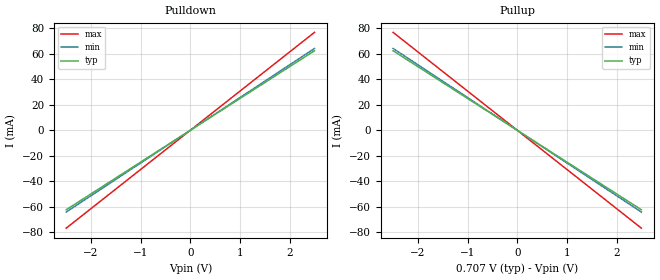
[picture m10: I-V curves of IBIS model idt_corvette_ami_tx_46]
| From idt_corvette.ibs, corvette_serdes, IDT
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|   model   idt_corvette_ami_tx_46
[Model] idt_corvette_ami_tx_46
Model_type Output
C_comp 400f 400f 400f
Cref = 0
[Model Spec]
Vmeas 0. 0. 0.
Vref 0. 0. 0.
[Temperature Range]  25 100 0
[Voltage Range] .707 .697 .631
[Algorithmic Model]
Executable Windows_VisualStudio5_32 idt_corvette_tx.dll   idt_corvette_tx.ami
Executable Windows_ver_64   idt_corvette_tx_64.dll   idt_corvette_tx.ami
Executable Linux_gcc4.1.2_32   idt_corvette_tx.linux.so   idt_corvette_tx.ami
Executable Linux_gcc3.2.3_64   idt_corvette_tx_64.linux.so idt_corvette_tx.ami
[End Algorithmic Model]
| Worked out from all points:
|   slope of the pulldown table from 0 to 0.106 V, typ, clamps not added: 40 ohm
|   slope of the pullup table from 0 to 0.106 V, typ, clamps not added: 40 ohm
[Pulldown]
-2.5V     -62.5mA    -64.31mA   -76.95mA
0V        0A         0A         0A
2.5V      62.5mA     64.31mA    76.95mA
[Pullup]
-2.5V     62.5mA     64.31mA    76.95mA
0V        0A         0A         0A
2.5V      -62.5mA    -64.31mA   -76.95mA
[Ramp]
dV/dt_r .236/22.4p .235/21.77p .229/18.194p
dV/dt_f .236/22.4p .235/21.77p .229/18.194p
